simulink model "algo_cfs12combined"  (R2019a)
settings: configuration reference "configurationSettings" (kept in a data dictionary, not in this file)
undefined symbols (not defined in the file or in its folder): algo_cfs1_fp, algo_cfs2_fp

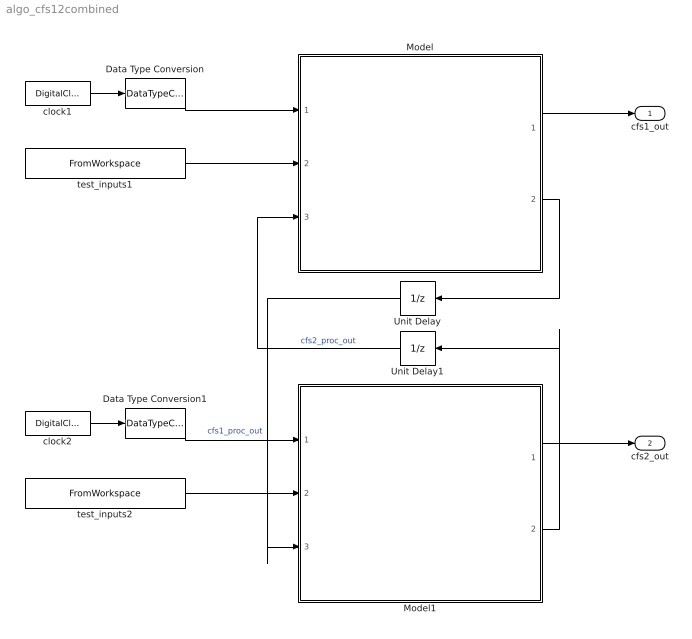
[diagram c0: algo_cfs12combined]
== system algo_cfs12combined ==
  Data Type Conversion : DataTypeConversion  OutDataTypeStr=single
  Data Type Conversion1 : DataTypeConversion  OutDataTypeStr=single
  Model : ModelReference  ModelNameDialog=algo_cfs1.slx  SimulationMode=Normal  ModelReferenceVersion=1.801  SimulationMode=Normal
  Model1 : ModelReference  ModelNameDialog=algo_cfs2.slx  SimulationMode=Normal  ModelReferenceVersion=1.795  SimulationMode=Normal
  Unit Delay : UnitDelay  SampleTime=-1  HasFrameUpgradeWarning=on
  Unit Delay1 : UnitDelay  SampleTime=-1  HasFrameUpgradeWarning=on
  clock1 : DigitalClock  SampleTime=algo_cfs1_fp.timing.dt
  clock2 : DigitalClock  SampleTime=algo_cfs1_fp.timing.dt
  test_inputs1 : FromWorkspace  VariableName=algo_cfs1_inbus1  OutDataTypeStr=Bus: algo_cfs1_inBus  SampleTime=algo_cfs1_fp.timing.dt  Interpolate=off  OutputAfterFinalValue=Holding final value
  test_inputs2 : FromWorkspace  VariableName=algo_cfs2_inbus1  OutDataTypeStr=Bus: algo_cfs2_inBus  SampleTime=algo_cfs2_fp.timing.dt  Interpolate=off  OutputAfterFinalValue=Holding final value
  cfs1_out : Outport  OutDataTypeStr=Bus: algo_cfs1_outBus
  cfs2_out : Outport  Port=2  OutDataTypeStr=Bus: algo_cfs2_outBus
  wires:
  Model1/2 -> Unit Delay1/1
  clock2/1 -> Data Type Conversion1/1
  Unit Delay1/1 -> Model/3  "cfs2_proc_out"
  Model1/1 -> cfs2_out/1
  Data Type Conversion1/1 -> Model1/1
  Model/1 -> cfs1_out/1
  test_inputs2/1 -> Model1/2
  Data Type Conversion/1 -> Model/1
  Model/2 -> Unit Delay/1
  Unit Delay/1 -> Model1/3  "cfs1_proc_out"
  test_inputs1/1 -> Model/2
  clock1/1 -> Data Type Conversion/1
